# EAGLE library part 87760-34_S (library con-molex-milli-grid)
HEADER
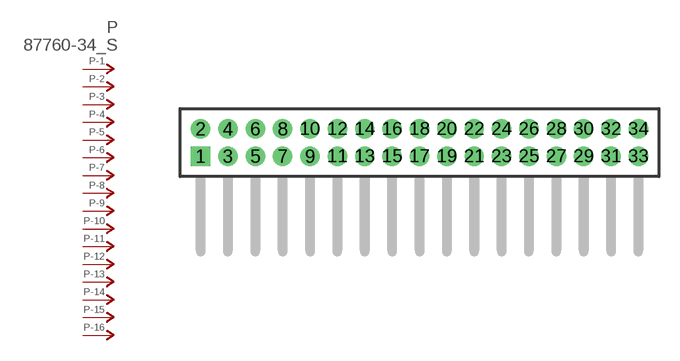
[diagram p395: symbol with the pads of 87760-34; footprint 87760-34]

Designator prefix P; gates -1=P-NV -2=P-N -3=P-N -4=P-N -5=P-N -6=P-N -7=P-N -8=P-N -9=P-N -10=P-N -11=P-N -12=P-N -13=P-N -14=P-N -15=P-N -16=P-N -17=P-N -18=P-N -19=P-N -20=P-N -21=P-N -22=P-N -23=P-N -24=P-N -25=P-N -26=P-N -27=P-N -28=P-N -29=P-N -30=P-N -31=P-N -32=P-N -33=P-N -34=P-N

## 87760-34_S  [87760-34]
1  -1:P  pas
2  -2:P  pas
3  -3:P  pas
4  -4:P  pas
5  -5:P  pas
6  -6:P  pas
7  -7:P  pas
8  -8:P  pas
9  -9:P  pas
10  -10:P  pas
11  -11:P  pas
12  -12:P  pas
13  -13:P  pas
14  -14:P  pas
15  -15:P  pas
16  -16:P  pas
17  -17:P  pas
18  -18:P  pas
19  -19:P  pas
20  -20:P  pas
21  -21:P  pas
22  -22:P  pas
23  -23:P  pas
24  -24:P  pas
25  -25:P  pas
26  -26:P  pas
27  -27:P  pas
28  -28:P  pas
29  -29:P  pas
30  -30:P  pas
31  -31:P  pas
32  -32:P  pas
33  -33:P  pas
34  -34:P  pas

## Footprint 87760-34 (pad centres in mm)
HEADER Dual Row, Right Angle
drill 0.914 square: 1 -16,-1
drill 0.914: 2 -16,1; 3 -14,-1; 4 -14,1; 5 -12,-1; 6 -12,1; 7 -10,-1; 8 -10,1; 9 -8,-1; 10 -8,1; 11 -6,-1; 12 -6,1; 13 -4,-1; 14 -4,1; 15 -2,-1; 16 -2,1; 17 0,-1; 18 0,1; 19 2,-1; 20 2,1; 21 4,-1; 22 4,1; 23 6,-1; 24 6,1; 25 8,-1; 26 8,1; 27 10,-1; 28 10,1; 29 12,-1; 30 12,1; 31 14,-1; 32 14,1; 33 16,-1; 34 16,1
